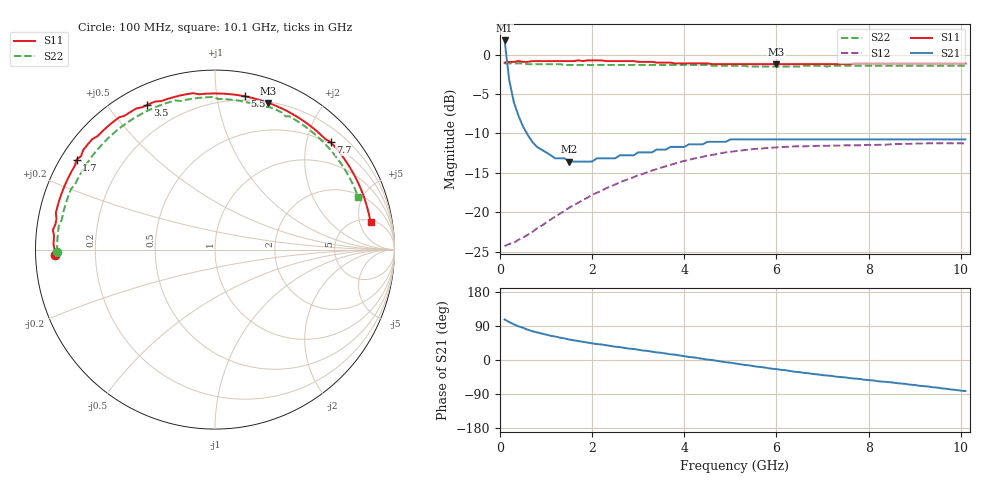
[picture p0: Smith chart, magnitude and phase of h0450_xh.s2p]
!HBFP-0450
!VC=.500V  IC=50.020mA  VB=.938 V  IB=734.980uA
# GHZ S MA R  50
!Measurement  Date:  23-Jul  1998  Time: 19:19:43
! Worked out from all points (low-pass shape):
!   101 points, 100 MHz to 10.1 GHz, reference 50 ohm
!   highest |S21| = 1.80 dB at 100 MHz (marker M1); lowest = -13.6 dB at 1.5 GHz (marker M2)
!   |S21| within 3 dB of the highest: start of sweep to 159.7 MHz
!   lowest |S11| = -1.2 dB at 6 GHz (marker M3), VSWR 14.38, Z = 10.5 + j70.4 ohm
!   |S11| at or under -10 dB: nowhere
!   |S22| runs from -1.5 to -1.1 dB; largest |S21 - S12| = 1.2
!   S11 on the Smith chart (normalised r, x): 100 MHz: 0.06, -0.02; 1.7 GHz: 0.05, +0.30; 3.5 GHz: 0.08, +0.63; 5.5 GHz: 0.17, +1.20; 7.7 GHz: 0.46, +2.46; 10.1 GHz: 5.48, +7.43
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0.1  0.89 -178.0  1.23 107.0  0.061 6.0  0.88 -179.0
0.2  0.9 178.0  0.69 100.0  0.063 9.0  0.88 178.0
0.3  0.9 175.0  0.5 94.0  0.064 12.0  0.88 175.0
0.4  0.91 173.0  0.41 89.0  0.067 15.0  0.88 173.0
0.6  0.9 169.0  0.31 80.0  0.072 18.0  0.87 169.0
0.8  0.91 164.0  0.26 73.0  0.079 23.0  0.87 166.0
1.2  0.91 156.0  0.22 62.0  0.094 27.0  0.87 158.0
1.5  0.91 151.0  0.21 54.0  0.107 28.0  0.86 153.0
1.7  0.92 147.0  0.21 50.0  0.115 27.0  0.86 150.0
1.8  0.91 145.0  0.21 48.0  0.12 27.0  0.86 148.0
2.1  0.92 140.0  0.22 42.0  0.133 26.0  0.86 144.0
2.8  0.91 127.0  0.23 30.0  0.163 20.0  0.86 133.0
3.5  0.89 115.0  0.25 19.0  0.192 12.0  0.86 122.0
4.4  0.88 99.0  0.27 3.0  0.225 -1.0  0.86 106.0
5.1  0.87 86.0  0.29 -9.0  0.244 -12.0  0.85 94.0
5.5  0.87 79.0  0.29 -16.0  0.252 -18.0  0.84 87.0
6  0.87 70.0  0.29 -24.0  0.258 -26.0  0.84 79.0
6.8  0.87 57.0  0.29 -37.0  0.263 -38.0  0.85 66.0
7.7  0.88 43.0  0.29 -49.0  0.266 -49.0  0.85 54.0
8.5  0.88 32.0  0.29 -59.0  0.27 -60.0  0.85 44.0
9.4  0.88 19.0  0.29 -72.0  0.274 -72.0  0.85 31.0
10.1  0.88 10.0  0.29 -82.0  0.273 -82.0  0.85 20.0
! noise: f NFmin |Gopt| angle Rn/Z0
1.8  3.32  0.91  -150  0.46
2  3.31  0.93  -146  0.63
2.5  3.27  0.87  -137  0.79
3.5  3.21  0.78  -122  0.98
4  3.17  0.77  -114  1.04
5  3.09  0.73  -96  1.33
5.5  2.88  0.76  -86  1.54
7  2.96  0.79  -59  2.27
8  2.8  0.72  -46  2.12
10  2.75  0.85  -14  3.49
